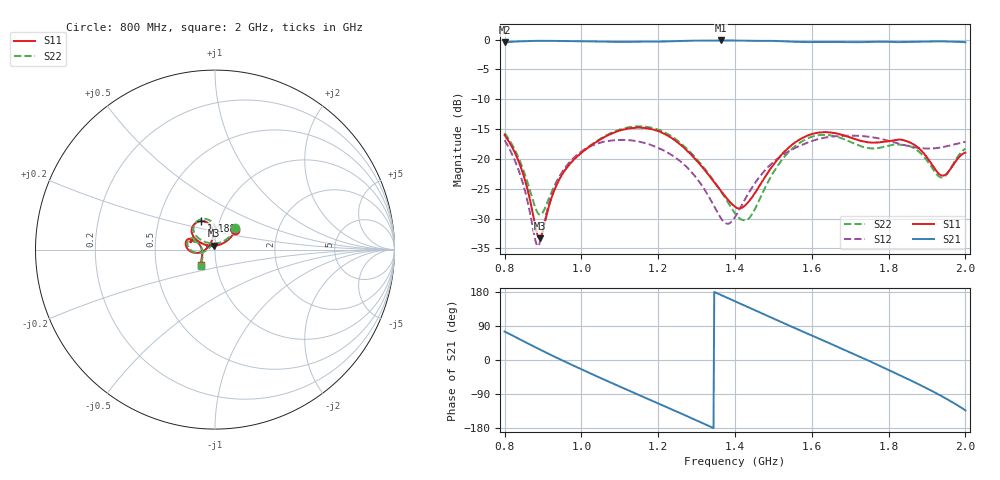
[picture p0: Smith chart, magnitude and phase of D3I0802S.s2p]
! 3/12/2021 10:51:04 AM
! C:\USERS\KOBYR\DESKTOP\0.8 - 2.0 GHZ (D3I0802N).S2P
! CHANNEL.1
! TR.MEASUREMENT
! CORRECTED.DATA
# GHZ S RI R 50.0
! FREQ.GHZ  S11RE  S11IM  S21RE  S21IM  S12RE  S12IM  S22RE  S22IM
!; PortSelection: Port_12
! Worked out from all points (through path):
!   601 points, 800 MHz to 2 GHz, reference 50 ohm
!   highest |S21| = -0.14 dB at 1.364 GHz (marker M1); lowest = -0.5 dB at 800 MHz (marker M2)
!   lowest |S11| = -33.3 dB at 892 MHz (marker M3), VSWR 1.04, Z = 49.6 + j2.11 ohm
!   |S11| at or under -10 dB: start of sweep to end of sweep
!   |S22| runs from -30.3 to -14.5 dB; largest |S21 - S12| = 1.1
!   S11 on the Smith chart (normalised r, x): 800 MHz: 1.22, +0.28; 1.188 GHz: 0.82, +0.27; 2 GHz: 0.85, -0.14
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0.8  0.1135 0.1103  0.2425 0.9168  0.0768 -0.1213  0.114 0.1187
0.842  0.069 0.0509  0.5807 0.7735  0.00898 -0.0708  0.0692 0.0611
0.88  0.0133 0.0238  0.8135 0.5399  0.00921 -0.0186  0.0149 0.036
0.892  -0.00372 0.0212  0.8663 0.4516  0.0184 -0.00806  -0.00148 0.0339
0.936  -0.0546 0.0274  0.9699 0.0989  0.0636 -0.00553  -0.0505 0.0414
1  -0.1003 0.0511  0.8814 -0.4023  0.0851 -0.078  -0.0939 0.0652
1.096  -0.1299 0.1121  0.3536 -0.8895  -0.0404 -0.1384  -0.119 0.1278
1.188  -0.0756 0.159  -0.3192 -0.9087  -0.1263 -0.0229  -0.0579 0.1715
1.2  -0.0651 0.1583  -0.4017 -0.8752  -0.1236 -0.00378  -0.0468 0.1698
1.288  -0.0111 0.1063  -0.8811 -0.4277  -0.0303 0.0706  0.00619 0.11
1.364  -0.0174 0.0508  -0.9729 0.1476  0.0302 0.00943  -0.00369 0.0531
1.4  -0.0275 0.0288  -0.8889 0.418  0.0154 -0.0287  -0.0148 0.0317
1.438  -0.0442 0.00773  -0.7226 0.6573  -0.0243 -0.0476  -0.0303 0.0112
1.504  -0.0915 -0.0175  -0.2966 0.9284  -0.0965 -0.00164  -0.079 -0.0178
1.6  -0.1606 0.0177  0.4026 0.8662  -0.0404 0.1354  -0.1519 0.0211
1.704  -0.1372 0.0599  0.9042 0.2951  0.1414 0.0677  -0.122 0.0629
1.756  -0.1285 0.0473  0.953 -0.093  0.1445 -0.0484  -0.1138 0.0451
1.8  -0.1348 0.041  0.8581 -0.4284  0.0721 -0.1225  -0.1236 0.0369
1.862  -0.1239 0.0512  0.5364 -0.7928  -0.0729 -0.1029  -0.1169 0.0446
1.912  -0.0861 0.028  0.1478 -0.9543  -0.121 0.017  -0.0821 0.0234
1.944  -0.0713 -0.0138  -0.145 -0.9545  -0.0775 0.0997  -0.0681 -0.0185
2  -0.076 -0.0835  -0.6486 -0.6954  0.1092 0.0867  -0.0782 -0.0934
